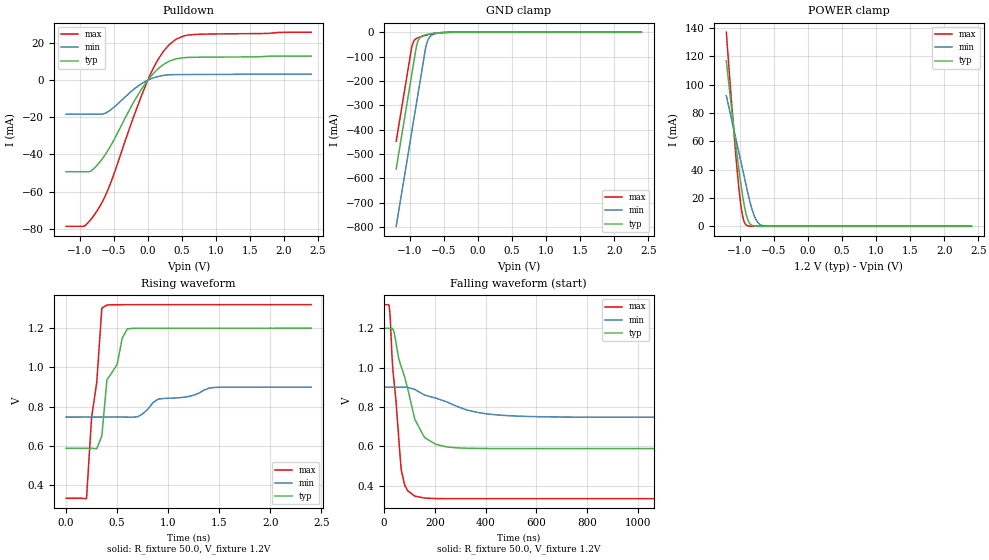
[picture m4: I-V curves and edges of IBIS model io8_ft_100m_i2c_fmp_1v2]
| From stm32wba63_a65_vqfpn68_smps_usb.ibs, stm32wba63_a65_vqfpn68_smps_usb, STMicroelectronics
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[Model]   io8_ft_100m_i2c_fmp_1v2
Model_type I/O_open_drain
Polarity   Non-Inverting
Enable   Active-Low
| CAP_THRESHOLD on pad IOFT is "UDTCAPC" :
| Rising=30.0% of vddiom   Falling=70.0% of vddiom
| C_comp min and max val. don't necessarily correlate with the min and max pvt
| but are the smallest and greatest pad capacitance found.
| var   typ   min   max
C_comp   2.87935pF  2.80370pF  2.98278pF
|C_comp_pulldown   2.87935pF  2.80370pF  2.98278pF
Vinl = 450.0mV
Vinh = 660.0mV
Vmeas = 600.0mV   | Reference voltage for timing measurements
Cref  = 50.0pF   | Timing specification test load capacitance value
Rref  = 1.0MOhm   | Timing specification test load resistance value
Vref  = 660.0mV   | Timing specification test load voltage
[Model Spec]
| TIME_THRESHOLD on pin ZII2CV11 is "CMOS" :
| Rising=50.0% of vdd   Falling=50.0% of vdd
Vinl 441.50000mV 335.50000mV 487.50000mV
Vinh 755.50000mV 552.50000mV 839.50000mV
| variable   typ   min   max
[Temperature Range] 25.0 140.0 -40.0
| variable   typ   min   max
[Voltage Range] 1.2V 900.0mV 1.32V
| variable   typ   min   max
[POWER Clamp Reference] 1.2V 900.0mV 1.32V
| variable   typ   min   max
[GND Clamp Reference] 0V 0V 0V
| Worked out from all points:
|   slope of the pulldown table from 0 to 0.18 V, typ, clamps not added: 25.7 ohm
|   GND clamp passes 1 mA (typ) near -0.51 V on its own axis
|   POWER clamp passes 1 mA (typ) near -0.83 V on its own axis
|   rising waveform, R_fixture 50.0, V_fixture 1.2V: 20-80 % time 163ps typ, 518ps min, 102ps max; typ from 0.588 V to 1.2 V
|   falling waveform, R_fixture 50.0, V_fixture 1.2V: 20-80 % time 78.4ns typ, 201ns min, 35.3ns max; typ from 1.2 V to 0.588 V
[POWER Clamp]
-1.2V     116.7mA    92.13mA    136.9mA
-1.09V    69.42mA    68.21mA    67.14mA
-1.02V    41.75mA    52.99mA    28.91mA
-990mV    30.98mA    46.47mA    16.09mA
-970mV    24.36mA    42.12mA    9.575mA
-940mV    15.59mA    35.6mA     3.485mA
-910mV    8.693mA    29.07mA    1.01mA
-860mV    2.259mA    18.59mA    104.6uA
-780mV    143.1uA    6.246mA    2.555uA
-720mV    16.22uA    1.846mA    157.1nA
-650mV    1.267uA    330.3uA    6.118nA
2.4V      0A         0A         0A
[GND Clamp]
-1.2V     -561.6mA   -797.4mA   -447.4mA
-980mV    -187.6mA   -423.4mA   -73.43mA
-960mV    -153.6mA   -389.4mA   -48.26mA
-900mV    -54.17mA   -287.4mA   -24.97mA
-870mV    -29.55mA   -236.4mA   -21.19mA
-830mV    -17.05mA   -168.4mA   -17.42mA
-760mV    -9.921mA   -54.55mA   -11.89mA
-730mV    -8.191mA   -29.78mA   -9.811mA
-690mV    -6.26mA    -14.49mA   -7.318mA
-600mV    -2.976mA   -4.315mA   -3.058mA
-380mV    -57.63uA   -251uA     -19.49uA
2.4V      872.8pA    204.8nA    349.4pA
| variable   typ   min   max
[Pullup Reference] 1.2V 900.0mV 1.32V
| variable   typ   min   max
[Pulldown Reference] 0V 0V 0V
[Pulldown]
-1.2V     -49.3mA    -18.35mA   -78.69mA
-930mV    -49.3mA    -18.35mA   -78.46mA
-830mV    -48.76mA   -18.35mA   -74.69mA
-700mV    -43.85mA   -18.35mA   -67.63mA
-540mV    -34.99mA   -15.84mA   -54.84mA
-200mV    -11.29mA   -4.684mA   -18.8mA
10mV      478.8uA    168.8uA    852.4uA
170mV     6.712mA    2.137mA    12.23mA
330mV     10.42mA    2.911mA    19.6mA
540mV     12.14mA    3.031mA    23.95mA
670mV     12.31mA    3.044mA    24.56mA
2.4V      12.92mA    3.23mA     25.77mA
[Ramp]
dV/dt_r 366.97414mV/3.28877ns 91.44519mV/10.33147ns 591.80329mV/1.7125ns
dV/dt_f 366.99015mV/75.86808ns 91.48132mV/200.55799ns 591.81478mV/34.98961ns
R_load = 50.0
| Removed startup time: 0s 0s 0s  .
| Removed end time: 2.4ns.
[Rising Waveform]
R_fixture   = 50.0
V_fixture   = 1.2V
V_fixture_min = 900.0mV
V_fixture_max = 1.32V
0s        588.3mV    747.5mV    333.6mV
200ps     588.3mV    747.5mV    331.5mV
250ps     588.4mV    747.5mV    747mV
300ps     585.7mV    747.5mV    923.3mV
350ps     651.2mV    747.5mV    1.302V
400ps     937.5mV    747.5mV    1.318V
500ps     1.016V     747.5mV    1.32V
600ps     1.197V     747.3mV    1.32V
1.4ns     1.2V       894.7mV    1.32V
2.4ns     1.2V       899.9mV    1.32V
| Removed startup time: 0s 0s 0s  .
| Removed end time: 1.99925us.
[Falling Waveform]
R_fixture   = 50.0
V_fixture   = 1.2V
V_fixture_min = 900.0mV
V_fixture_max = 1.32V
0s        1.2V       900mV      1.32V
22.25ns   1.2V       900mV      1.294V
34.5ns    1.197V     900mV      1.001V
68.75ns   1.002V     900mV      476.3mV
93ns      894.4mV    899.6mV    374.4mV
122.5ns   734.2mV    888mV      346.4mV
163.3ns   641.6mV    859.2mV    336.6mV
285.8ns   592.1mV    803.6mV    333.7mV
571.3ns   588.4mV    751.5mV    333.6mV
1.999us   588.3mV    747.5mV    333.6mV
